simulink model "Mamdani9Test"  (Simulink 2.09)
settings: Solver=ode45  StartTime=0.0  StopTime=10  MaxStep=10  RelTol=1e-3  AbsTol=1e-3
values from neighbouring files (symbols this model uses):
  k_s = 1.1    [Mdata.m]    (also in Mdata25.m)
  tau = 1    [Mdata.m]    (also in Mdata25.m; VdataC.m = m/kv)
  yd = 1    [Mdata.m]    (also in Mdata25.m)
undefined symbols (not defined in the file or in its folder): sfunyst
libraries: fuzzy x2

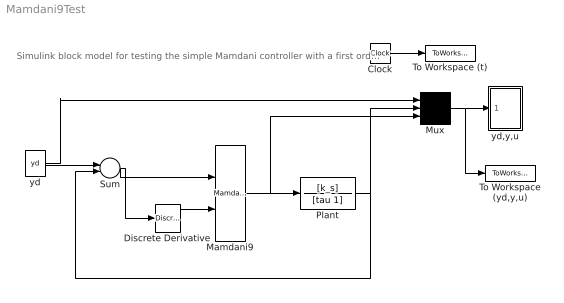
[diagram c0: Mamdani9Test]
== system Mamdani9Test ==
  note: Simulink block model for testing the simple Mamdani controller with a first order plan
  Clock : Clock
  Discrete Derivative : fuzzy/Discrete Derivative
  Mamdani9 : fuzzy/Mamdani9
  Mux : Mux  Inputs=3
  Plant : TransferFcn  Numerator=[k_s]  Denominator=[tau 1]
  Sum : Sum  Inputs=+-
  To Workspace (yd,y,u) : ToWorkspace  VariableName=yout  SampleTime=0
  To Workspace (t) : ToWorkspace  VariableName=t  SampleTime=0
  yd : Constant  Value=yd
  yd,y,u : Subsystem  mask(Storage scope.){}
      mask help: Storage scope using MATLAB graph window. Enter plotting ranges and line type.
      mask init:
      | npts = @4; color = @5; ax = [0, @1, @2, @3]; dt=-1;
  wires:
  Mux/1 -> yd,y,u/1(x), To Workspace (yd,y,u)/1
  yd/1 -> Mux/1, Sum/1
  Mamdani9/1 -> Plant/1, Mux/3
  Discrete Derivative/1 -> Mamdani9/2
  Sum/1 -> Discrete Derivative/1, Mamdani9/1
  Plant/1 -> Mux/2, Sum/2
  Clock/1 -> To Workspace (t)/1

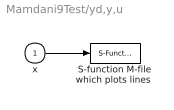
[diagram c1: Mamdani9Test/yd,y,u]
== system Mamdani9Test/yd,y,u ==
  x : Inport  Port=1  PortWidth=-1  SampleTime=-1
  "S-function M-file which plots lines " : S-Function  LoadFcn=sfunyst([],[],[],'LoadBlock')  FunctionName=sfunyst  Parameters=ax, color, npts, dt
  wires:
  x/1 -> "S-function M-file which plots lines "/1
